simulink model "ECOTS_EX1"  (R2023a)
settings: Solver=ode23tb  StartTime=0.0  StopTime=meas.Time(end)  RelTol=1e-3
libraries: component_lib x3

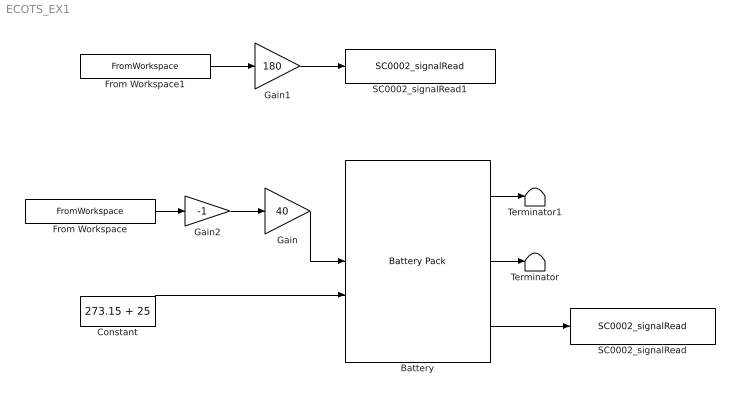
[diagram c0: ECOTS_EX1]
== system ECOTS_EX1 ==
  Battery : component_lib/Battery Pack  SOC_0=1  Nx=40  Ny=180
  Constant : Constant  Value=273.15 + 25
  From Workspace : FromWorkspace  VariableName=[meas.Time, meas.Current]
  From Workspace1 : FromWorkspace  VariableName=[meas.Time, meas.Voltage]
  Gain : Gain  Gain=40
  Gain1 : Gain  Gain=180
  Gain2 : Gain  Gain=-1
  SC0002_signalRead : component_lib/Data & Control/SC0002_signalRead  SigName=generatedHeat
  SC0002_signalRead1 : component_lib/Data & Control/SC0002_signalRead  SigName=measuredBatteryVoltage
  Terminator : Terminator
  Terminator1 : Terminator
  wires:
  Constant/1 -> Battery/2
  Battery/2 -> Terminator/1
  Battery/1 -> Terminator1/1
  Battery/3 -> SC0002_signalRead/1
  From Workspace/1 -> Gain2/1
  Gain/1 -> Battery/1
  Gain1/1 -> SC0002_signalRead1/1
  From Workspace1/1 -> Gain1/1
  Gain2/1 -> Gain/1
